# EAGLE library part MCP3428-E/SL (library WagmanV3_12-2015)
Analog-to-Digital Converter
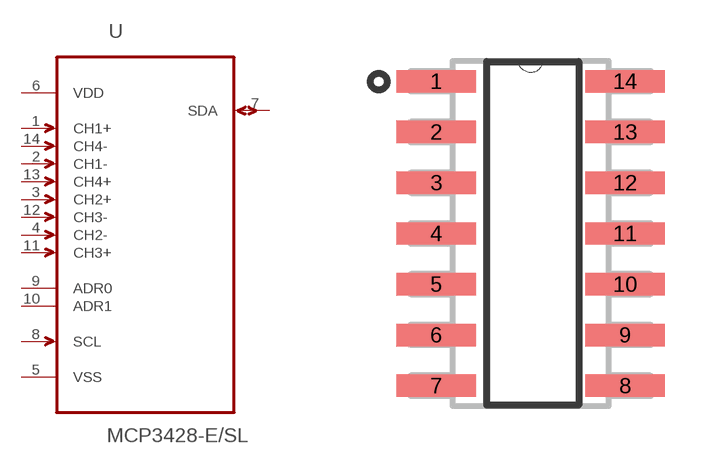
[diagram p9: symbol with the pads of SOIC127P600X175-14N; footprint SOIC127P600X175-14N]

Designator prefix -

## MCP3428-E/SL (MPN: MCP3428-E/SL; OC_FARNELL: 1825014; OC_NEWARK: 52R9962; PACKAGE: SOIC-14; SUPPLIER: Microchip)  [SOIC127P600X175-14N]
1  CH1+  in
2  CH1-  in
3  CH2+  in
4  CH2-  in
5  VSS  pwr
6  VDD  pwr
7  SDA
8  SCL  in
9  ADR0  pas
10  ADR1  pas
11  CH3+  in
12  CH3-  in
13  CH4+  in
14  CH4-  in

## Footprint SOIC127P600X175-14N (pad centres in mm)
smd 1.981 x 0.559: 1 -2.362,3.81; 2 -2.362,2.54; 3 -2.362,1.27; 4 -2.362,0; 5 -2.362,-1.27; 6 -2.362,-2.54; 7 -2.362,-3.81; 8 2.362,-3.81; 9 2.362,-2.54; 10 2.362,-1.27; 11 2.362,0; 12 2.362,1.27; 13 2.362,2.54; 14 2.362,3.81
